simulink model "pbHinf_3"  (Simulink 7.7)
settings: Solver=ode45  StartTime=0.0  StopTime=10.0  RelTol=1e-3
libraries: cstblocks x3

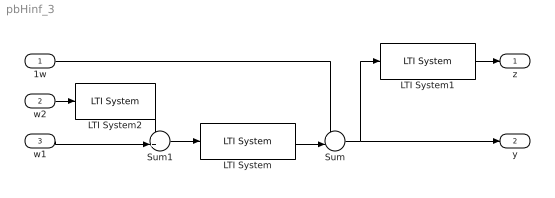
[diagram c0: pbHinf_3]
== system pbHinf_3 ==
  1w : Inport
  w2 : Inport  Port=2
  w1 : Inport  Port=3
  LTI System : cstblocks/LTI System  SystemSampleTime=-1  sys=G  IC=[]
  LTI System1 : cstblocks/LTI System  SystemSampleTime=-1  sys=W1  IC=[]
  LTI System2 : cstblocks/LTI System  SystemSampleTime=-1  sys=W2  IC=[]
  Sum : Sum  Inputs=+-|
  Sum1 : Sum  Inputs=++|
  z : Outport
  y : Outport  Port=2
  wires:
  LTI System/1 -> Sum/2
  1w/1 -> Sum/1
  LTI System1/1 -> z/1
  Sum/1 -> y/1, LTI System1/1
  w1/1 -> Sum1/2
  Sum1/1 -> LTI System/1
  w2/1 -> LTI System2/1
  LTI System2/1 -> Sum1/1
